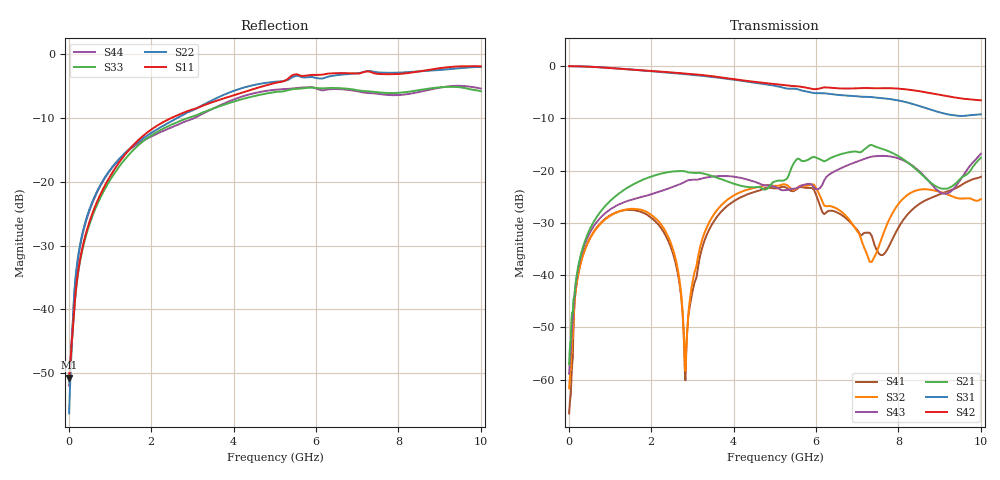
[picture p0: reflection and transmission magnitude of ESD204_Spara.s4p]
! Created Thu Apr  5 15:26:45 2018
# hz S ma R 50
! 4 Port Network Data from SP1.SP block
! freq  magS11  angS11  magS12  angS12  magS13  angS13  magS14  angS14
!  magS21  angS21  magS22  angS22  magS23  angS23  magS24  angS24
!  magS31  angS31  magS32  angS32  magS33  angS33  magS34  angS34
!  magS41  angS41  magS42  angS42  magS43  angS43  magS44  angS44
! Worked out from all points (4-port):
!   1000 points, 10 MHz to 10 GHz, reference 50 ohm
!   strongest paths, dB at 10 MHz, 2.51 GHz, 5.01 GHz, 7.51 GHz, 10 GHz:
!     S42: 0.0, -1.2, -3.4, -4.2, -6.5
!     S31: 0.0, -1.3, -3.8, -6.1, -9.2
!     S21: -57.0, -20.2, -22.1, -15.6, -17.5
!     S43: -58.8, -23.1, -23.1, -17.2, -16.8
!     S32: -61.6, -34.6, -22.9, -34.8, -25.4
!     S41: -66.4, -35.4, -23.4, -35.7, -21.2
!   lowest |S11| = -50.7 dB at 10 MHz (marker M1), VSWR 1.01, Z = 50.1 - j0.282 ohm
!   |S11| at or under -10 dB: start of sweep to 2.505 GHz
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1e7  0.002921 -74.6  0.0008361 -90.4  0.999 -0.3  0.000518 166.6
     0.001406 177.7  0.001541 -122.6  0.0007213 145.6  1.002 -0.4
     0.9998 -0.3  0.0008281 22.4  0.00272 -99.0  0.001269 -97.7
     0.0004774 176.9  1 -0.3  0.001146 65.2  0.002525 -125.8
1.03e9  0.1136 26.2  0.05247 173.6  0.9613 -7.6  0.03799 55.8
        0.05246 173.5  0.1267 33.2  0.03752 60.7  0.9585 -8.8
        0.9612 -7.6  0.03748 60.7  0.1061 105.3  0.04325 -48.3
        0.03788 55.8  0.9585 -8.8  0.0432 -48.1  0.1254 99.9
2.83e9  0.3514 -116.6  0.09868 -34.5  0.8378 -20.2  0.0008556 123.9
        0.09848 -34.5  0.3409 -125.2  0.001116 -84.7  0.8491 -21.7
        0.8378 -20.1  0.001215 -84.7  0.3096 -140.0  0.07864 141.1
        0.0009893 124.8  0.8496 -21.7  0.07874 141.2  0.2957 -132.9
4e9  0.4736 19.4  0.07542 55.6  0.7423 -27.7  0.05096 -157.6
     0.07528 55.6  0.512 21.9  0.05776 -166.6  0.7513 -28.1
     0.7426 -27.7  0.05784 -166.6  0.4223 63.2  0.08771 19.2
     0.05094 -157.6  0.7516 -28.1  0.08769 19.2  0.4384 68.8
7.13e9  0.7153 11.1  0.1551 -67.4  0.5109 -35.9  0.02457 -138.3
        0.1549 -67.4  0.7184 7.4  0.02002 121.2  0.6177 -42.6
        0.5105 -35.9  0.02015 121.0  0.5124 32.3  0.1281 123.1
        0.02467 -138.0  0.6184 -42.6  0.1281 123.1  0.4993 52.8
8.55e9  0.7316 -174.5  0.09324 68.6  0.4109 -28.2  0.04925 -20.1
        0.09314 68.7  0.7299 -157.2  0.06604 5.4  0.5715 -40.4
        0.4109 -28.1  0.0662 5.4  0.5224 -178.5  0.09508 -38.5
        0.04923 -20.3  0.5727 -40.5  0.09507 -38.5  0.5068 -150.7
1e10  0.7966 2.0  0.1332 128.6  0.3461 0.2  0.08735 11.1
      0.1329 128.5  0.7895 12.1  0.05366 56.0  0.4711 -42.1
      0.3462 0.2  0.05363 55.8  0.5098 -24.3  0.1455 -113.0
      0.08734 11.1  0.472 -42.2  0.1452 -112.9  0.5339 18.5
